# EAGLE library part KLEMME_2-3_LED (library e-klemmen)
Dreistock-Initiatoren-Klemme mit LED
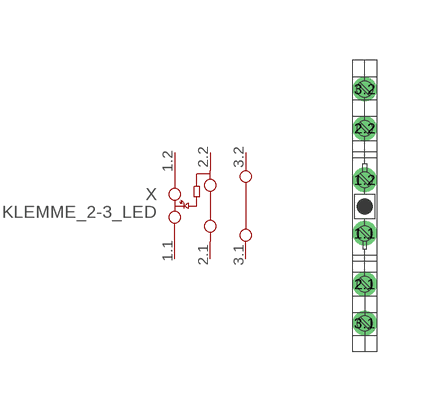
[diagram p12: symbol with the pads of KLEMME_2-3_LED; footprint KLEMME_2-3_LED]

Designator prefix X

## KLEMME_2-3_LED  [KLEMME_2-3_LED]
1.1  1.1  pas
1.2  1.2  pas
2.1  2.1  pas
2.2  2.2  pas
3.1  3.1  pas
3.2  3.2  pas

## Footprint KLEMME_2-3_LED (pad centres in mm)
Dreistock-Initiatoren-Klemme, Querschnitt: 0,2 - 2,5 mm², AWG: 30 - 14, Breite: 6,2 mm, Farbe: grau Quelle: http://download.phoenixcontact.de .. c2715814.dxf
drill 0.1 pad 0.2: 1.1 0,-0.67; 1.2 0,0.67; 2.1 0,-1.94; 2.2 0,1.96; 3.1 0,-2.92; 3.2 0,2.94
